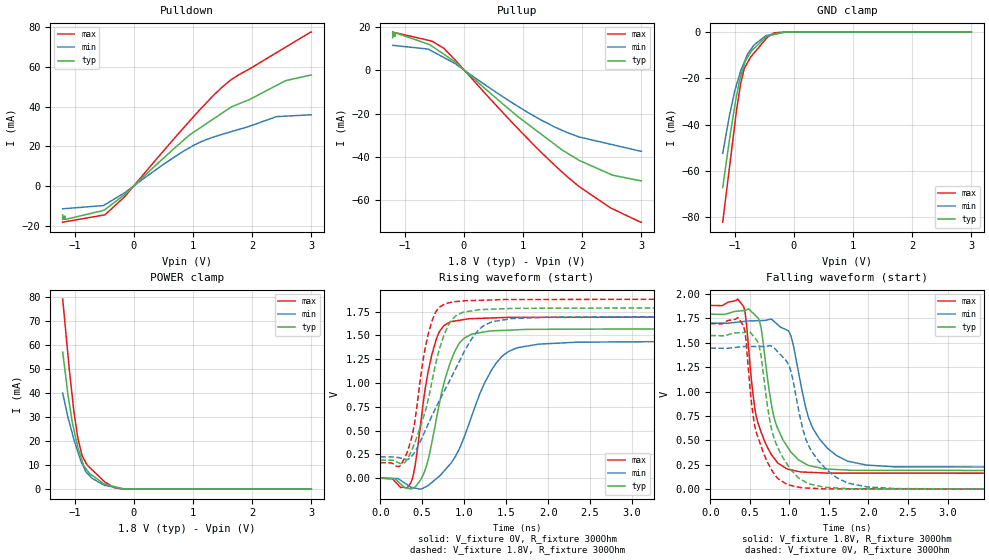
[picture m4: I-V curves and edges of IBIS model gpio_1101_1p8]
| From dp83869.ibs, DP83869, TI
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|   gpio_1101_1p8 Model
[Model]   gpio_1101_1p8
Model_type   I/O
Polarity   Non-Inverting
Enable   Active-Low
Vinl = 0.344
Vinh = 1.204
Vmeas = 0.9
Vref = 0
Cref = 2pF
Rref = 100000
|   typ   min   max
C_comp   1.311pF   1.163pF   1.492pF
| Where Nom  PVT is Nominal Process, 1.8V,  27C
|   Fast PVT is Strong Process,  1.89V, -40C
|   Slow PVT is Weak Process,   1.71V, 125C
[Voltage Range]   1.8   1.71   1.89
|Junction Temperature
[Temperature Range]   27   125   -40
[Pullup Reference]   1.8   1.71   1.89
[Pulldown Reference]   0   -0   -0
[Power Clamp Reference]   1.8   1.71   1.89
[GND Clamp Reference]   0   0   0
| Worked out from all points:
|   slope of the pulldown table from 0 to 0.27 V, typ, clamps not added: 35.6 ohm
|   slope of the pullup table from 0 to 0.27 V, typ, clamps not added: 41.4 ohm
|   GND clamp passes 1 mA (typ) near -0.32 V on its own axis
|   POWER clamp passes 1 mA (typ) near -0.31 V on its own axis
|   falling waveform, V_fixture 1.8V, R_fixture 300Ohm: 20-80 % time 243ps typ, 310ps min, 205ps max; typ from 1.79 V to 0.19 V
|   rising waveform, V_fixture 0V, R_fixture 300Ohm: 20-80 % time 253ps typ, 409ps min, 185ps max; typ from 0 V to 1.57 V
|   rising waveform, V_fixture 1.8V, R_fixture 300Ohm: 20-80 % time 281ps typ, 503ps min, 186ps max; typ from 0.19 V to 1.79 V
|   falling waveform, V_fixture 0V, R_fixture 300Ohm: 20-80 % time 267ps typ, 334ps min, 220ps max; typ from 1.57 V to 0 V
[Pulldown]
|   Voltage   I(typ)   I(min)   I(max)
-1.2V     -14.67mA   -11.53mA   -18.29mA
-1.199V   -16.94mA   -11.53mA   -18.28mA
-1.176V   -15.27mA   -11.48mA   -18.16mA
-1.173V   -16.82mA   -11.47mA   -18.14mA
-1.161V   -15.24mA   -11.44mA   -18.08mA
-1.133V   -16.74mA   -11.37mA   -17.94mA
-485.7mV  -11.91mA   -9.42mA    -14.56mA
-149.8mV  -4.276mA   -3.396mA   -5.332mA
835.9mV   22.96mA    17.45mA    29.12mA
1.479V    36.44mA    25.91mA    49.46mA
2.41V     50.69mA    34.97mA    67.21mA
3V        55.93mA    35.89mA    77.62mA
[GND Clamp]
|   Voltage   I(typ)   I(min)   I(max)
-1.2V     -67.24mA   -52.42mA   -82.2mA
-1.087V   -46.78mA   -36.13mA   -58.7mA
-994.5mV  -31.71mA   -25.26mA   -39.62mA
-964.6mV  -27.31mA   -22.67mA   -33.43mA
-896.5mV  -19mA      -16.78mA   -22.29mA
-837.6mV  -14.12mA   -13.07mA   -15.88mA
-780mV    -10.95mA   -9.493mA   -13.18mA
-671.1mV  -7.102mA   -5.59mA    -9.083mA
-440.9mV  -1.677mA   -1.364mA   -2.103mA
-325.9mV  -1.015mA   -827.4uA   -283.9uA
-149.8mV  -2.235uA   -5.466uA   -2.282uA
3V        0A         0A         0A
[Pullup]
|   Voltage   I(typ)   I(min)   I(max)
-1.2V     14.88mA    11.42mA    17.53mA
-1.199V   17.47mA    11.42mA    17.53mA
-1.176V   15.55mA    11.36mA    17.38mA
-1.173V   17.28mA    11.35mA    17.36mA
-1.163V   15.51mA    11.32mA    17.3mA
-1.147V   17.15mA    11.27mA    17.2mA
-603mV    12mA       9.72mA     13.79mA
-341.9mV  7.433mA    5.907mA    10.17mA
835.9mV   -19.59mA   -15.36mA   -24.66mA
1.66V     -36.74mA   -27.69mA   -46.95mA
2.515V    -48.4mA    -34.37mA   -63.92mA
3V        -50.97mA   -37.36mA   -70.05mA
[POWER Clamp]
|   Voltage   I(typ)   I(min)   I(max)
-1.2V     57.06mA    40.03mA    79.18mA
-1.112V   39.49mA    30mA       56.03mA
-1.038V   27.79mA    23.21mA    38.38mA
-1.012V   24.89mA    20.81mA    32.45mA
-946.5mV  17.68mA    15.73mA    21.61mA
-873.2mV  11.92mA    10.65mA    13.96mA
-845.4mV  9.816mA    9.19mA     12.7mA
-786.5mV  7.829mA    6.671mA    10.03mA
-492mV    2.077mA    1.583mA    3.049mA
-321.5mV  1.043mA    798.5uA    551.7uA
-149.8mV  3.268uA    8.848uA    3.514uA
3V        0A         0A         0A
[Ramp]
R_load = 300
|   typ   min   max
dV/dt_r   0.94405/2.51435e-10   0.866493/4.08512e-10   1.01734/1.83796e-10
dV/dt_f   0.961703/2.42785e-10   0.88705/3.08103e-10   1.03207/2.04368e-10
[Falling Waveform]
V_fixture = 1.8V
V_fixture_min = 1.71V
V_fixture_max = 1.89V
R_fixture = 300Ohm
C_fixture = 0F
|   Time   V(typ)   V(min)   V(max)
0s        1.793V     1.702V     1.883V
422.5ps   1.829V     1.719V     1.869V
541.7ps   1.803V     1.725V     959.6mV
605.5ps   1.753V     1.726V     673.7mV
796ps     771.3mV    1.725V     329.4mV
964.5ps   448.2mV    1.632V     209.4mV
1.047ns   357mV      1.487V     193.1mV
1.286ns   235.2mV    643.1mV    171.6mV
1.729ns   195.8mV    290mV      164.7mV
5ns       189.7mV    223.6mV    162.4mV
[Rising Waveform]
V_fixture = 0V
V_fixture_min = 0V
V_fixture_max = 0V
R_fixture = 300Ohm
C_fixture = 0F
|   Time   V(typ)   V(min)   V(max)
0s        73.36uV    183.5uV    51.44uV
365ps     -113mV     -95.25mV   -44.58mV
419ps     -88.62mV   -105.2mV   154.6mV
508.6ps   29.49mV    -105.8mV   770.6mV
612.3ps   363.2mV    -46.3mV    1.289V
831.1ps   1.208V     146.7mV    1.642V
999.2ps   1.472V     431.8mV    1.668V
1.316ns   1.548V     1.121V     1.684V
1.614ns   1.559V     1.365V     1.69V
5ns       1.573V     1.444V     1.696V
[Rising Waveform]
V_fixture = 1.8V
V_fixture_min = 1.71V
V_fixture_max = 1.89V
R_fixture = 300Ohm
C_fixture = 0F
|   Time   V(typ)   V(min)   V(max)
0s        189.7mV    223.6mV    162.4mV
228.1ps   157mV      213.8mV    122.5mV
307.9ps   182.8mV    196.9mV    244.6mV
404.5ps   357.5mV    266mV      559.7mV
577.6ps   851.4mV    582.3mV    1.535V
770.8ps   1.527V     930.5mV    1.832V
900.2ps   1.706V     1.153V     1.856V
1.126ns   1.763V     1.511V     1.868V
1.343ns   1.777V     1.646V     1.874V
5ns       1.793V     1.702V     1.883V
[Falling Waveform]
|Gnd
V_fixture = 0V
V_fixture_min = 0V
V_fixture_max = 0V
R_fixture = 300Ohm
C_fixture = 0F
|   Time   V(typ)   V(min)   V(max)
0s        1.574V     1.445V     1.696V
421ps     1.605V     1.462V     1.672V
450.1ps   1.608V     1.462V     1.534V
526.2ps   1.587V     1.462V     848.9mV
598.4ps   1.512V     1.462V     541.4mV
775ps     610.8mV    1.464V     196.8mV
970.5ps   257.3mV    1.302V     48.2mV
1.258ns   52.62mV    422.2mV    10.2mV
1.729ns   6.345mV    65.56mV    2.611mV
5ns       72.89uV    180.6uV    51.38uV
